(* Logix 5000 AddOnInstructionDefinition export AMCI_3601_AOP_Manual_Move_CCW; software revision 20.03 *)

ADD_ON_INSTRUCTION AMCI_3601_AOP_Manual_Move_CCW   (* revision 0.0, vendor AMCI, ExecuteEnableInFalse *)
// Revision note:
// 3/2020: Version 0 is the initial release
VAR_INPUT
   Axis_Status_Bits : INT; {required}
   _0_normal_1_S_Curve_Acceleration : BOOL;
   _0_Triangular_1_Trapezoidal_S_Curve : BOOL;
   Programmed_Speed : DINT; {required}
   Acceleration : INT; {required}
   Deceleration : INT; {required}
END_VAR
VAR_OUTPUT
   EN : BOOL; {access Read Only, visible}
   Manual_Move_CCW_Occurring : BOOL; {access Read Only, visible}
   ER : BOOL; {access Read Only, visible}
END_VAR
VAR_IN_OUT
   AMCI_3601_output_data : AM:1769_3601:O:0; {required}
END_VAR
VAR
   Upper_Result_X_1000 : DINT;
   command_data_block : INT[10];
        [0]   // Command Bits MSW
        [1]   // Command Bits LSW
        [2]   // Upper Target Position
        [3]   // Lower Target Position
        [4]   // Upper Programmed Speed
        [5]   // Lower Programmed Speed
END_VAR

ROUTINE EnableInFalse   (* ladder *)
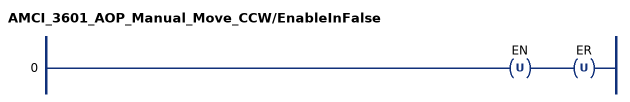
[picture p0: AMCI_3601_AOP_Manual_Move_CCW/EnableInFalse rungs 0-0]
   0: OTU(EN)OTU(ER);
END_ROUTINE

ROUTINE Logic   (* ladder *)
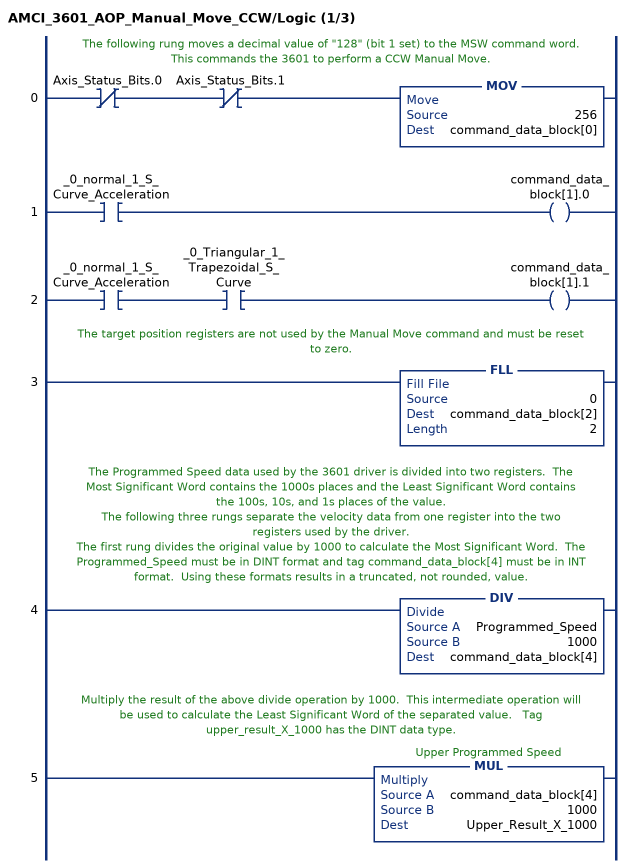
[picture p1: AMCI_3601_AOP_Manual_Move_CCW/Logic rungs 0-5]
   // The following rung moves a decimal value of "128" (bit 1 set) to the MSW command word.  This commands the 3601 to perform a CCW Manual Move.
   0: XIO(Axis_Status_Bits.0)XIO(Axis_Status_Bits.1)MOV(256,command_data_block[0]);
   1: XIC(_0_normal_1_S_Curve_Acceleration)OTE(command_data_block[1].0);
   2: XIC(_0_normal_1_S_Curve_Acceleration)XIC(_0_Triangular_1_Trapezoidal_S_Curve)OTE(command_data_block[1].1);
   // The target position registers are not used by the Manual Move command and must be reset to zero.
   3: FLL(0,command_data_block[2],2);
   // The Programmed Speed data used by the 3601 driver is divided into two registers.  The Most Significant Word contains the 1000s places and the Least Significant Word contains the 100s, 10s, and 1s places of the value.
   // The following three rungs separate the velocity data from one register into the two registers used by the driver.
   // The first rung divides the original value by 1000 to calculate the Most Significant Word.  The Programmed_Speed must be in DINT format and tag command_data_block[4] must be in INT format.  Using these formats results in a truncated, not rounded, value.
   4: DIV(Programmed_Speed,1000,command_data_block[4]);
   // Multiply the result of the above divide operation by 1000.  This intermediate operation will be used to calculate the Least Significant Word of the separated value.   Tag upper_result_X_1000 has the DINT data type.
   5: MUL(command_data_block[4],1000,Upper_Result_X_1000);
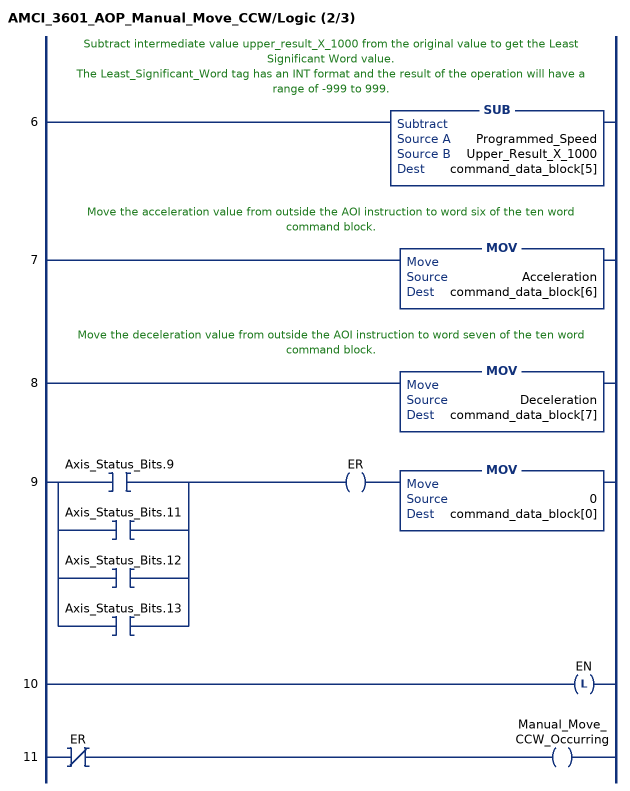
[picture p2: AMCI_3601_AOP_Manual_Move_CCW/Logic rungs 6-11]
   // Subtract intermediate value upper_result_X_1000 from the original value to get the Least Significant Word value.
   // The Least_Significant_Word tag has an INT format and the result of the operation will have a range of -999 to 999.
   6: SUB(Programmed_Speed,Upper_Result_X_1000,command_data_block[5]);
   // Move the acceleration value from outside the AOI instruction to word six of the ten word command block.
   7: MOV(Acceleration,command_data_block[6]);
   // Move the deceleration value from outside the AOI instruction to word seven of the ten word command block.
   8: MOV(Deceleration,command_data_block[7]);
   9: [XIC(Axis_Status_Bits.9) ,XIC(Axis_Status_Bits.11) ,XIC(Axis_Status_Bits.12) ,XIC(Axis_Status_Bits.13) ]OTE(ER)MOV(0,command_data_block[0]);
   10: OTL(EN);
   11: XIO(ER)OTE(Manual_Move_CCW_Occurring);
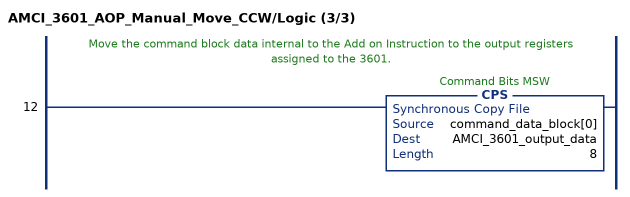
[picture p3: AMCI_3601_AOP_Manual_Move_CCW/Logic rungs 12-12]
   // Move the command block data internal to the Add on Instruction to the output registers assigned to the 3601.
   12: CPS(command_data_block[0],AMCI_3601_output_data,8);
END_ROUTINE
END_ADD_ON_INSTRUCTION
